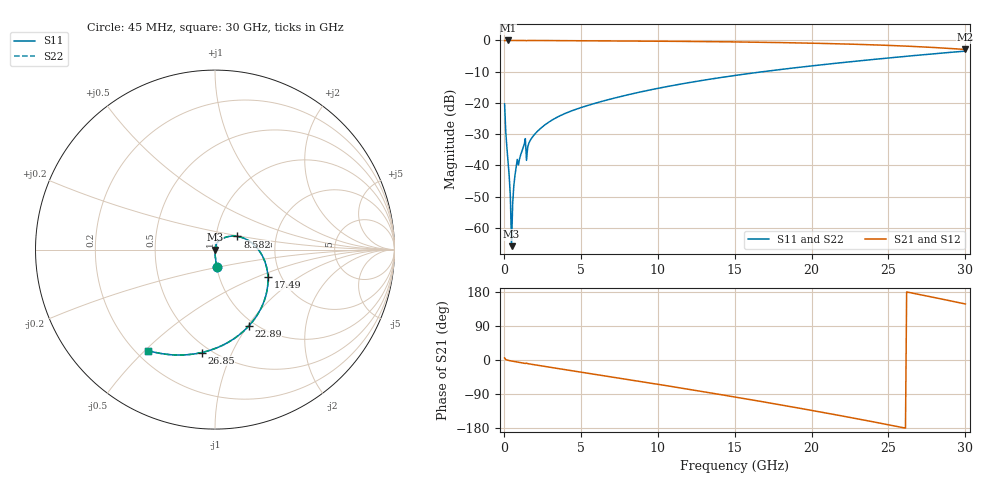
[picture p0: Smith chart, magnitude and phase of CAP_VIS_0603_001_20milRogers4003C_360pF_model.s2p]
! S-parameter model data by Modelithics Inc.  support@modelithics.com  813-866-6335  Tampa FL USA
! S-Parameter data specifications:
! Substrate: 20-mil Rogers 4003C, substrate thickness, H=0.508mm, Dielectric constant, Er=3.75
! PCB Mounting Pad Footprint: Pad width, PadW=0.90mm , Pad length, PadL=1.00mm , Pad gap, PadG (edge-to-edge)=1.00mm , Reference planes=3.0mm apart
! Created Wed Nov 18 13:34:13 2015
# hz S ma R 50
! 2 Port Network Data from SP1.SP block
! freq  magS11  angS11  magS21  angS21  magS12  angS12  magS22  angS22
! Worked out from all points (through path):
!   401 points, 45 MHz to 30 GHz, reference 50 ohm
!   highest |S21| = 0.00 dB at 269.7 MHz (marker M1); lowest = -2.9 dB at 30 GHz (marker M2)
!   group delay of S21, straight-line fit = 19.4 ps
!   lowest |S11| = -65.8 dB at 494.3 MHz (marker M3), VSWR 1.00, Z = 50 - j0.0199 ohm
!   |S11| at or under -10 dB: start of sweep to 16.83 GHz
!   |S22| runs from -65.8 to -3.4 dB; largest |S21 - S12| = 0
!   S11 on the Smith chart (normalised r, x): 45 MHz: 1.00, -0.19; 8.582 GHz: 1.27, +0.19; 17.49 GHz: 1.71, -0.58; 22.89 GHz: 0.93, -1.01; 26.85 GHz: 0.45, -0.77; 30 GHz: 0.25, -0.51
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4.5e7  0.09676 -84.6  0.9951 5.3  0.9951 5.3  0.09676 -84.6
1.94775e8  0.01923 -89.0  0.9995 0.0  0.9995 0.0  0.01923 -89.0
2.696625e8  0.01163 -89.0  0.9995 -0.8  0.9995 -0.8  0.01163 -89.0
3.4455e8  0.006755 -88.0  0.9995 -1.5  0.9995 -1.5  0.006755 -88.0
4.94325e8  0.0005121 -22.9  0.9995 -2.7  0.9995 -2.7  0.0005121 -22.9
6.441e8  0.004728 79.5  0.9994 -3.8  0.9994 -3.8  0.004728 79.5
7.189875e8  0.006942 80.6  0.9993 -4.3  0.9993 -4.3  0.006942 80.6
7.93875e8  0.009263 80.4  0.9991 -4.8  0.9991 -4.8  0.009263 80.4
1.2432e9  0.01902 79.3  0.9988 -7.8  0.9988 -7.8  0.01902 79.3
1.617638e9  0.02261 77.0  0.9984 -10.1  0.9984 -10.1  0.02261 77.0
1.992075e9  0.03142 74.8  0.9979 -12.6  0.9979 -12.6  0.03142 74.8
2.890725e9  0.04887 67.8  0.9954 -18.5  0.9954 -18.5  0.04887 67.8
5.062462e9  0.08516 51.4  0.9866 -32.3  0.9866 -32.3  0.08516 51.4
8.582175e9  0.1445 30.6  0.9771 -54.8  0.9771 -54.8  0.1445 30.6
1.007992e10  0.1727 21.5  0.9721 -64.5  0.9721 -64.5  0.1727 21.5
1.50225e10  0.2754 -10.3  0.9472 -97.7  0.9472 -97.7  0.2754 -10.3
1.749379e10  0.3315 -27.2  0.9285 -114.9  0.9285 -114.9  0.3315 -27.2
2.003996e10  0.3926 -45.2  0.9038 -133.2  0.9038 -133.2  0.3926 -45.2
2.288569e10  0.4659 -66.3  0.8678 -154.5  0.8678 -154.5  0.4659 -66.3
2.505742e10  0.5259 -83.1  0.8323 -171.4  0.8323 -171.4  0.5259 -83.1
2.685472e10  0.5785 -97.4  0.7965 174.1  0.7965 174.1  0.5785 -97.4
3e10  0.6752 -123.6  0.7165 147.8  0.7165 147.8  0.6752 -123.6
